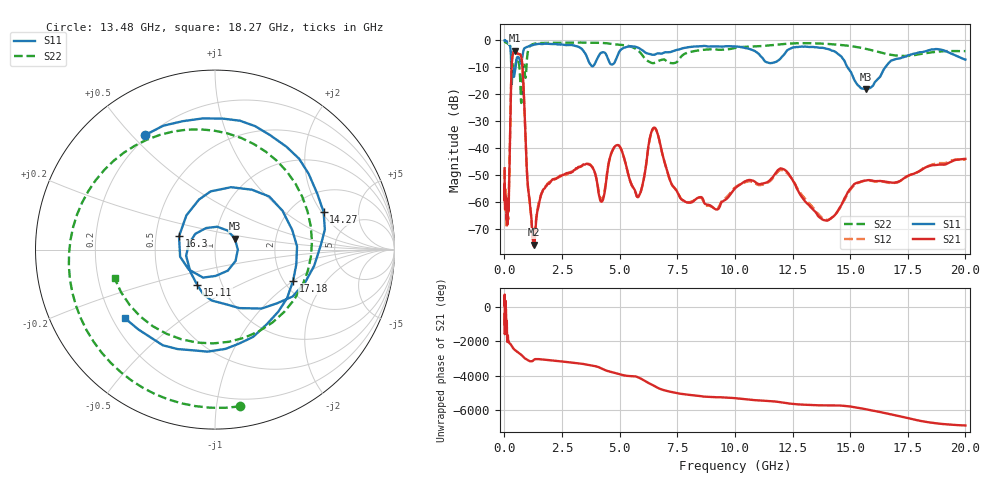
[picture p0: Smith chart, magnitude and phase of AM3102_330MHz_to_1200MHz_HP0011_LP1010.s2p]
! Date/Time: Tue, Sep 11, 2018 5:12 PM
! Network Analyzer: Agilent Technologies E8362B Rev: A.07.50.63
! Sweep from 0.010 to 20.000 GHz, 1601 Points, Sweep Type: LOG
! Power Supply: 4.949 V, 0.001 A
# Hz S DB R 50
!freq MagS11 AngS11 MagS21 AngS21 MagS12 AngS12 MagS22 AngS22
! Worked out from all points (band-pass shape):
!   1601 points, 10 MHz to 20 GHz, reference 50 ohm
!   highest |S21| = -3.72 dB at 447.2 MHz (marker M1); lowest = -75.6 dB at 1.266 GHz (marker M2)
!   |S21| within 3 dB of the highest: 336.7 MHz to 746.2 MHz (409.5 MHz wide, 75.6 % of centre)
!   lowest |S11| = -18.0 dB at 15.7 GHz (marker M3), VSWR 1.29, Z = 61.9 + j7.61 ohm
!   |S11| at or under -10 dB: 299 MHz to 482.6 MHz (183.7 MHz wide, 47 % of centre); 14.89 GHz to 16.52 GHz (1.626 GHz wide, 10.4 % of centre)
!   |S22| runs from -23.2 to -0.3 dB; largest |S21 - S12| = 0.012
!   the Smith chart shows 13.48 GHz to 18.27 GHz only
!   S11 on the Smith chart (normalised r, x): 13.48 GHz: 0.19, +0.55; 14.27 GHz: 2.96, +2.10; 15.11 GHz: 0.76, -0.31; 16.3 GHz: 0.66, +0.10; 17.18 GHz: 2.23, -1.00; 18.27 GHz: 0.25, -0.32
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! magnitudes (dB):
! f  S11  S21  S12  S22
! 10 MHz  0.0  -47.4  -48.3  -0.3
! 35.55 MHz  0.0  -60.5  -61.2  -0.5
! 126.4 MHz  -0.4  -67.5  -64.5  -1.0
! 184.8 MHz  -1.0  -61.9  -59.8  -1.3
! 313.2 MHz  -15.4  -9.8  -9.9  -5.4
! 447.2 MHz  -12.0  -3.7  -3.8  -10.5
! 765 MHz  -6.8  -8.1  -8.1  -18.2
! 1.266 GHz  -1.6  -75.6  -76.2  -1.3
! 1.59 GHz  -1.3  -57.3  -57.1  -0.9
! 4.23 GHz  -4.4  -59.7  -59.0  -0.9
! 4.878 GHz  -6.3  -38.8  -38.8  -1.5
! 5.652 GHz  -2.3  -55.3  -55.7  -2.9
! 6.518 GHz  -5.3  -32.3  -32.5  -8.3
! 7.845 GHz  -2.7  -59.8  -59.7  -4.8
! 13.48 GHz  -2.5  -63.4  -63.1  -1.1
! 14.27 GHz  -3.9  -65.2  -65.2  -1.4
! 15.11 GHz  -13.2  -53.9  -54.2  -2.2
! 15.7 GHz  -18.0  -51.9  -51.9  -3.1
! 16.3 GHz  -13.4  -52.1  -52.2  -4.4
! 17.18 GHz  -6.6  -52.0  -52.0  -5.7
! 18.27 GHz  -4.0  -47.0  -47.0  -4.7
! 20 GHz  -7.1  -43.9  -44.2  -3.9
